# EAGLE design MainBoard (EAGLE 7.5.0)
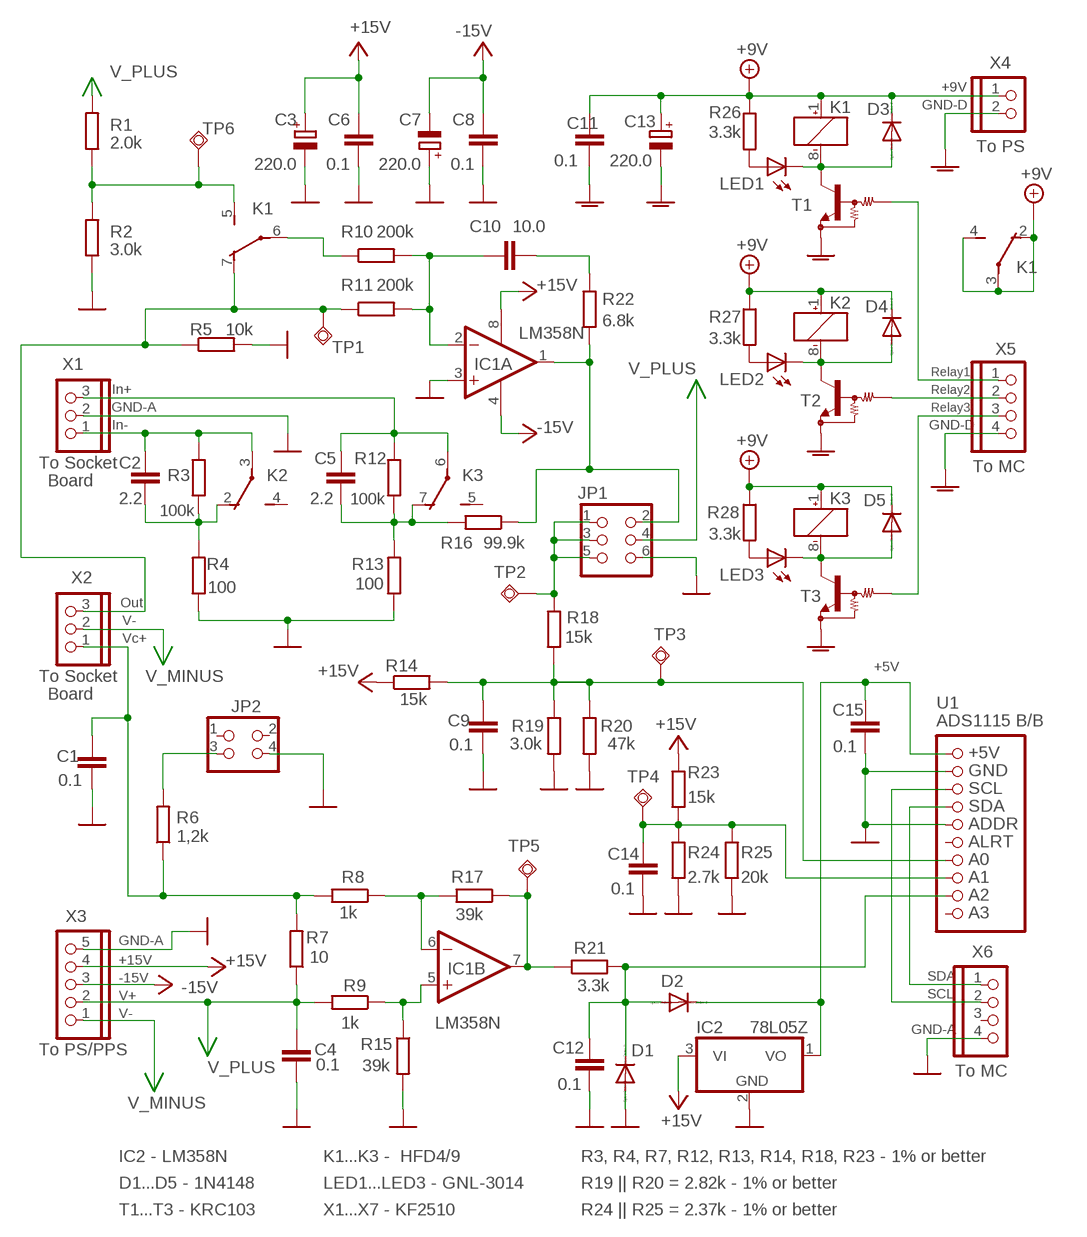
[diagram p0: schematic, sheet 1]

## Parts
C1  0.1  C-EU050-025X075  [C050-025X075]
C2  2.2  C-EU050-025X075  [C050-025X075]
C3  220.0  CPOL-EUE3.5-8  [E3,5-8]
C4  0.1  C-EU075-032X103  [C075-032X103]
C5  2.2  C-EU050-025X075  [C050-025X075]
C6  0.1  C-EU050-025X075  [C050-025X075]
C7  220.0  CPOL-EUE2.5-6  [E2,5-6]
C8  0.1  C-EU050-025X075  [C050-025X075]
C9  0.1  C-EU050-025X075  [C050-025X075]
C10  10.0  C-EU050-025X075  [C050-025X075]
C11  0.1  C-EU050-025X075  [C050-025X075]
C12  0.1  C-EU050-025X075  [C050-025X075]
C13  220.0  CPOL-EUE5-8.5  [E5-8,5]
C14  0.1  C-EU050-025X075  [C050-025X075]
C15  0.1  C-EU050-025X075  [C050-025X075]
D1  1N4148  DIODE-D-5  [D-5]
D2  1N4148  DIODE-D-5  [D-5]
D3  1N4148  DIODE-D-5  [D-5]
D4  1N4148  DIODE-D-5  [D-5]
D5  1N4148  DIODE-D-5  [D-5]
IC1  LM358N  [DIL08]
IC2  78L05Z  [TO92]
JP1  Dupont 2x3  PINHD-2X3  [2X03]
JP2  Dupont 2x2  PINHD-2X2  [2X02]
K1  GQ20009  [GQ]
K2  GQ20009  [GQ]
K3  GQ20009  [GQ]
LED1  GNL-3014  LED3MM  [LED3MM]
LED2  GNL-3014  LED3MM  [LED3MM]
LED3  GNL-3014  LED3MM  [LED3MM]
R1  2.0k  R-EU_0204/7  [0204/7]
R2  3.0k  R-EU_0204/5  [0204/5]
R3  100k  R-EU_0204/5  [0204/5]
R4  100  R-EU_0204/5  [0204/5]
R5  10k  R-EU_0204/7  [0204/7]
R6  1,2k  R-EU_0204/5  [0204/5]
R7  10  R-EU_0204/5  [0204/5]
R8  1k  R-EU_0204/5  [0204/5]
R9  1k  R-EU_0204/5  [0204/5]
R10  200k  R-EU_0204/5  [0204/5]
R11  200k  R-EU_0204/5  [0204/5]
R12  100k  R-EU_0204/5  [0204/5]
R13  100  R-EU_0204/5  [0204/5]
R14  15k  R-EU_0204/5  [0204/5]
R15  39k  R-EU_0204/5  [0204/5]
R16  99.9k  R-EU_0204/7  [0204/7]
R17  39k  R-EU_0204/5  [0204/5]
R18  15k  R-EU_0204/7  [0204/7]
R19  3.0k  R-EU_0204/5  [0204/5]
R20  47k  R-EU_0204/5  [0204/5]
R21  3.3k  R-EU_0204/5  [0204/5]
R22  6.8k  R-EU_0204/5  [0204/5]
R23  15k  R-EU_0204/5  [0204/5]
R24  2.7k  R-EU_0204/5  [0204/5]
R25  20k  R-EU_0204/5  [0204/5]
R26  3.3k  R-EU_0204/5  [0204/5]
R27  3.3k  R-EU_0204/5  [0204/5]
R28  3.3k  R-EU_0204/5  [0204/5]
T1  KRC103  -NPN_DRIVER-TO-92  [TO92-ECB]
T2  KRC103  -NPN_DRIVER-TO-92  [TO92-ECB]
T3  KRC103  -NPN_DRIVER-TO-92  [TO92-ECB]
TP1  TPSQPAD1-13  [P1-13]
TP2  TPSQPAD1-13  [P1-13]
TP3  TPSQPAD1-13  [P1-13]
TP4  TPSQPAD1-13  [P1-13]
TP5  TPSQPAD1-13  [P1-13]
TP6  TPSQPAD1-13  [P1-13]
U1  ADS1115 B/B  PINHD-1X10  [1X10]
X1  KF2510-3P  PINHD-1X3  [1X03]
X2  KF2510-3P  PINHD-1X3  [1X03]
X3  KF2510-5P  PINHD-1X5  [1X05]
X4  KF2510-2P  PINHD-1X2  [1X02]
X5  KF2510-4P  PINHD-1X4  [1X04]
X6  KF2510-4P  PINHD-1X4  [1X04]

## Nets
+5V: C15.2 D2.C IC2.1(VO) U1.1
+9V: C11.2 C13.+ D3.C D4.C D5.C K1.1(1:+) K1.2(2:O) K1.3(2:P) K1.4(2:S) K2.1(1:+) K3.1(1:+) R26.1 R27.1 R28.1 X4.1
ADC_A0: C9.2 R14.2 R18.2 R19.1 R20.1 TP3.TP U1.7
GND-A: C1.1 C3.- C4.1 C6.1 C7.+ C8.1 C9.1 C12.1 C14.1 C15.1 D1.A IC1.3(A:+IN) IC2.2(GND) JP1.6 JP2.4 R2.1 R4.1 R5.2 R13.1 R15.2 R19.2 R20.2 R24.2 R25.2 U1.2 U1.5 X1.2 X3.5 X6.4 ; supply symbol labelled GND
GND-D: C11.1 C13.- T1.E T2.E T3.E X4.2 X5.4 ; supply symbol labelled GNDA
N$1: C2.1 K2.2(2:O) R3.1 R4.2
N$2: C5.1 K3.7(3:O) R12.1 R13.2 R16.2
N$3: C2.2 K2.3(2:P) R3.2 X1.1
N$4: C5.2 K3.6(3:P) R12.2 X1.3
N$5: C14.2 R23.2 R24.1 R25.1 TP4.TP U1.8
N$6: D3.A K1.8(1:-) LED1.K(C) T1.C
N$7: T2.B X5.2
N$9: K1.6(3:P) R10.1
N$11: C10.1 IC1.2(A:-IN) R10.2 R11.2
N$12: C10.2 R22.1
N$13: D4.A K2.8(1:-) LED2.K(C) T2.C
N$14: IC1.7(B:OUT) R17.1 R21.1 TP5.TP
N$15: LED3.A R28.2
N$16: D5.A K3.8(1:-) LED3.K(C) T3.C
N$17: LED2.A R27.2
N$18: JP2.3 R6.2
N$19: K1.5(3:S) R1.1 R2.2 TP6.TP
N$22: T1.B X5.1
N$23: T3.B X5.3
N$24: IC1.6(B:-IN) R8.1 R17.2
N$25: LED1.A R26.2
N$26: IC1.5(B:+IN) R9.1 R15.1
N$27: IC1.1(A:OUT) JP1.2 R16.1 R22.2
N$28: U1.3 X6.2
N$29: U1.4 X6.1
N$31: JP1.1 JP1.3 JP1.5 R18.1 TP2.TP
N$35: C12.2 D1.C D2.A R21.2 U1.9
OUT: K1.7(3:O) R5.1 R11.1 TP1.TP X2.3
V+: C3.+ C6.2 IC1.8(P:V+) IC2.3(VI) R14.1 R23.1 X3.4 ; supply symbol labelled +15V
V-: C7.- C8.2 IC1.4(P:V-) X3.3 ; supply symbol labelled -15V
V_MINUS: X2.2 X3.1
V_PLUS: C4.2 JP1.4 R1.2 R7.1 R9.2 X3.2
VC_PLUS: C1.2 R6.1 R7.2 R8.2 X2.1
Unconnected: JP2.1 JP2.2 K2.4(2:S) K2.5(3:S) K2.6(3:P) K2.7(3:O) K3.2(2:O) K3.3(2:P) K3.4(2:S) K3.5(3:S) U1.6 U1.10 X6.3

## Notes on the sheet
- +9V
- GND-D
- To PS
- Relay1
- In+ | Relay2
- GND-A | Relay3
- In- | GND-D
- To MC
- To Socket
- Board
- Out
- V-
- Vc+
- +5V
- To Socket
- Board
- +5V
- GND
- SCL
- SDA
- ADDR
- ALRT
- A0
- A1
- A2
- A3
- GND-A
- +15V
- -15V | SDA
- V+ | SCL
- V-
- GND-A
- To PS/PPS
- To MC
- IC2 - LM358N | K1...K3 -  HFD4/9 | R3, R4, R7, R12, R13, R14, R18, R23 - 1% or better
- D1...D5 - 1N4148 | LED1...LED3 - GNL-3014 | R19 || R20 = 2.82k - 1% or better
- T1...T3 - KRC103 | X1...X7 - KF2510 | R24 || R25 = 2.37k - 1% or better

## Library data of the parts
C1 C2 C4-C6 C8-C12 C14 C15 = resistor:C-EU: CAPACITOR, European symbol
C3 C7 C13 = resistor:CPOL-EU: POLARIZED CAPACITOR, European symbol
D1-D5 = diode:DIODE-: DIODE
IC1 = linear:LM358: OP AMP also LM158; LM258; LM2904 Source: http://cache.national.com/ds/LM/LM158.pdf
IC2 = linear:78*: Positive VOLTAGE REGULATOR Source: http://cache.national.com/ds/LM/LM78L05.pdf http://www.fairchildsemi.com/ds/LM/LM7805.pdf
JP1 = pinhead:PINHD-2X3: PIN HEADER
JP2 = pinhead:PINHD-2X2: PIN HEADER
K1-K3 = relay:GQ?*: ULTRA-SMALL PACKAGE FLAT POLARIZED RELAY NAiS Source: http://www.mew-europe.com/.. en_ds_61008_0000.pdf; MF: AROMAT/ MATSUSHITA; MPN: AGQ20009; OC_FARNELL: unknown; OC_NEWARK: 10C3361
LED1-LED3 = led:LED: LED
R1-R28 = resistor:R-EU_: RESISTOR, European symbol
T1-T3 = transistor-neu-to92:*-NPN_DRIVER-: NPN Bias Resistor Transistor
TP1-TP6 = testpad:TPSQ: Test pad
U1 = pinhead:PINHD-1X10: PIN HEADER
X1 X2 = pinhead:PINHD-1X3: PIN HEADER
X3 = pinhead:PINHD-1X5: PIN HEADER
X4 = pinhead:PINHD-1X2: PIN HEADER
X5 X6 = pinhead:PINHD-1X4: PIN HEADER

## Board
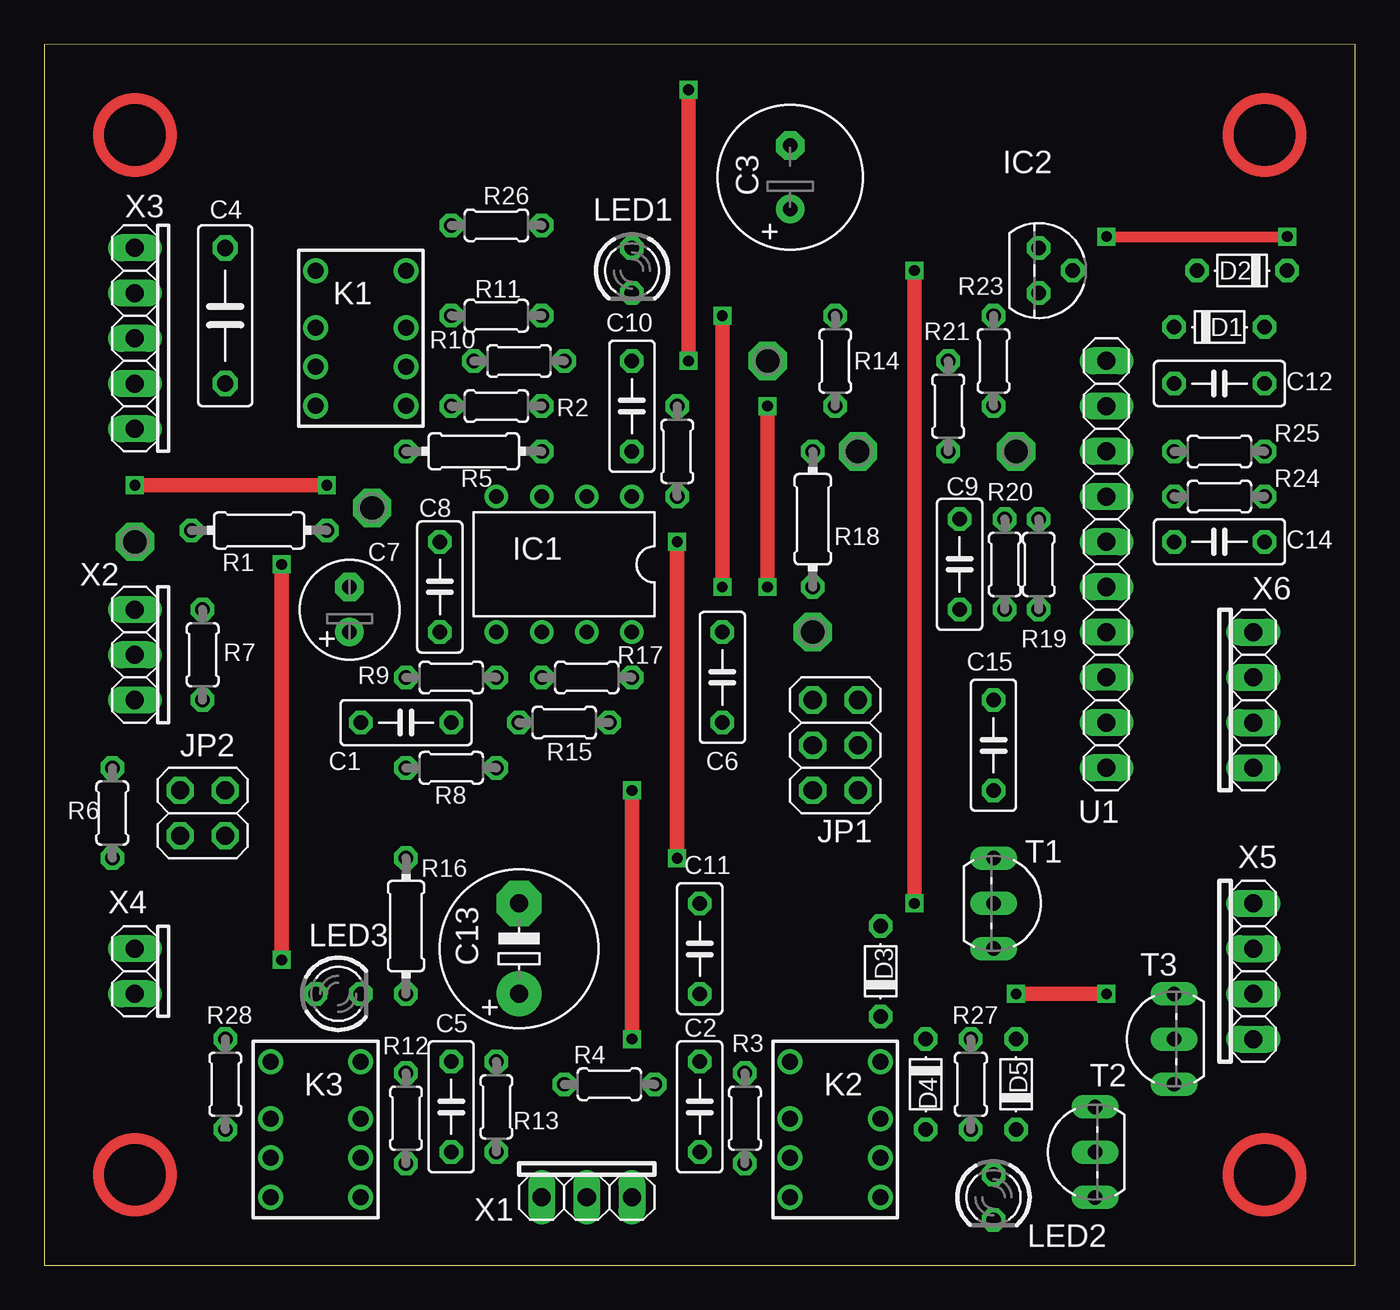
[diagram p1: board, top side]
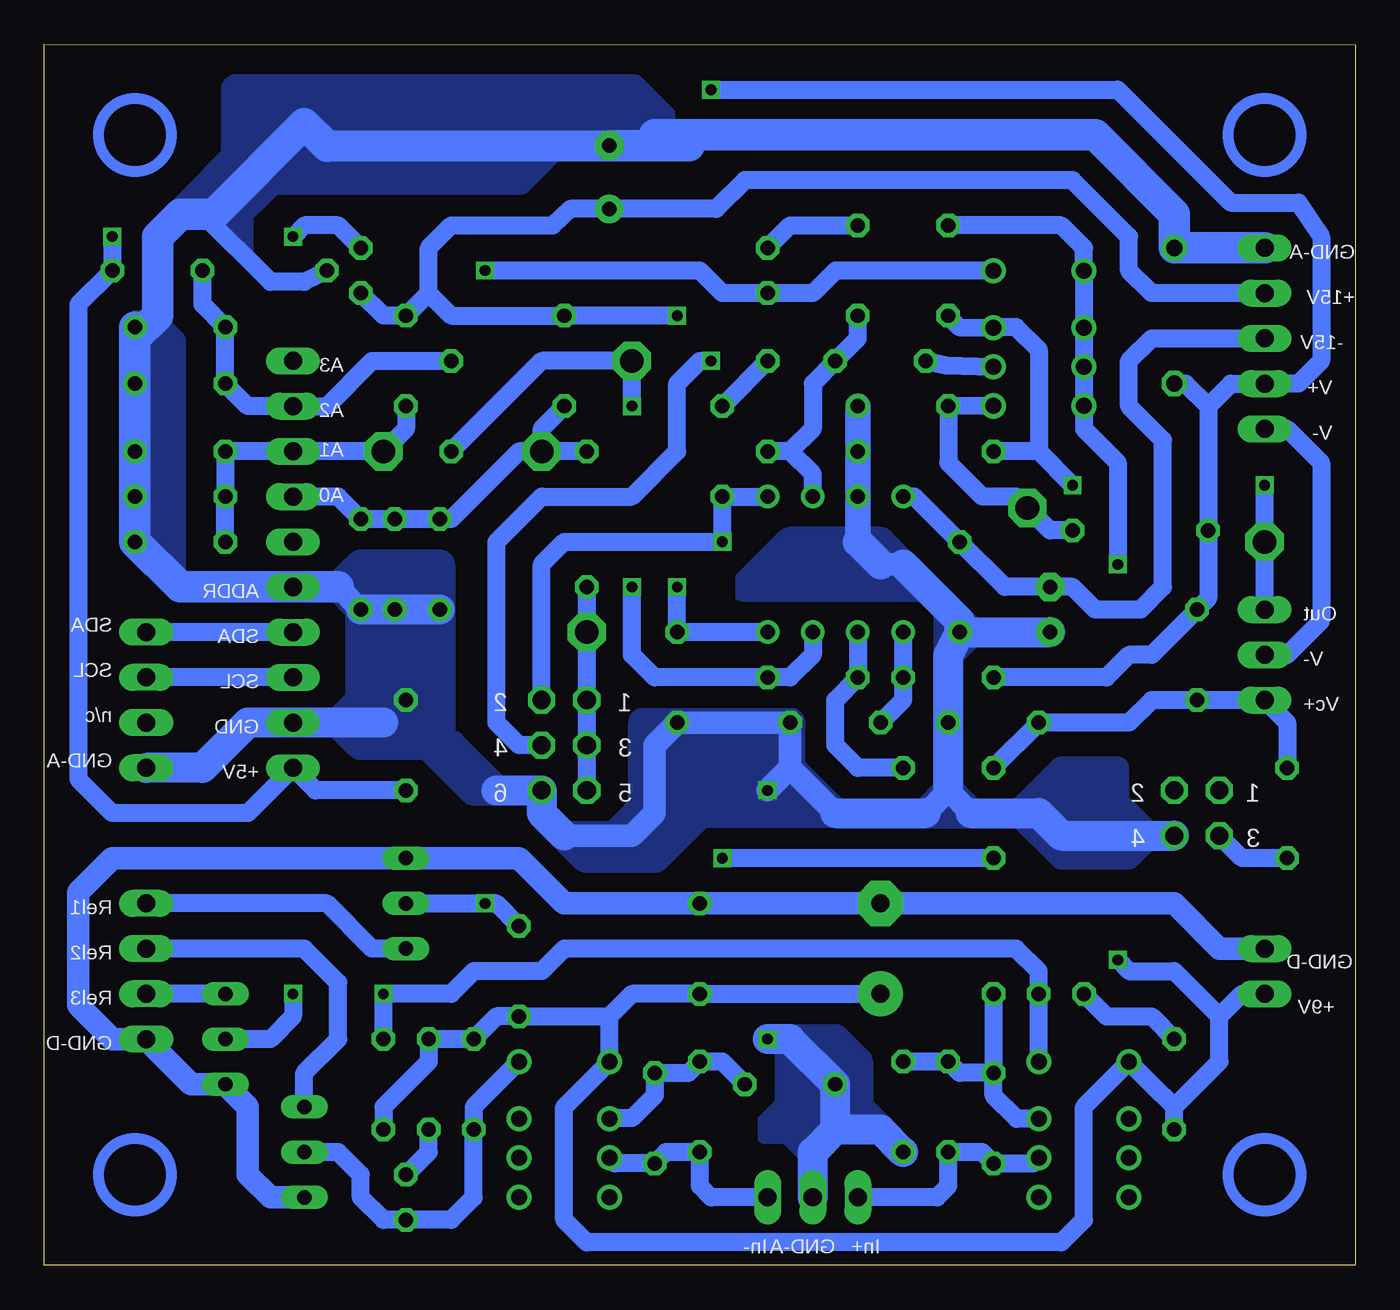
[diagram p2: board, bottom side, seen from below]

Size 73.66 x 68.58 mm. Coordinates in mm from the lower left corner, seen from the top.
Outline: 0,0 73.66,0 73.66,68.58 0,68.57 0,0
Copper layers (1*16): Top 0.035mm / dielectric 1.5mm / Bottom 0.035mm
Design rules "default *": minimum track width 10mil, minimum drill 10mil, track to track 8mil, track to pad 8mil, pad to pad 8mil, via to via 8mil, smd to smd 0mil, copper to edge 0mil, drill to drill 0mil, minimum pad ring 10mil, minimum via ring 8mil, stop-mask expansion 4mil, vias tented up to drill 0mil, thermal gap 10mil

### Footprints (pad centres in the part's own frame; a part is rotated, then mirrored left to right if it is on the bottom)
C050-025X075 = drill 0.813 octagon: 1 -2.54,0; 2 2.54,0
E3,5-8 = drill 0.813 pad 1.6: + -1.778,0 | drill 0.813 pad 1.6 octagon: - 1.778,0
C075-032X103 = drill 0.914 octagon: 1 -3.81,0; 2 3.81,0
E2,5-6 = drill 0.813 pad 1.6: + -1.27,0 | drill 0.813 pad 1.6 octagon: - 1.27,0
E5-8,5 = drill 1.016 pad 2.54: + -2.54,0 | drill 1.016 pad 2.54 octagon: - 2.54,0
D-5 = drill 0.813 octagon: A 2.54,0; C -2.54,0
DIL08 = drill 0.813 pad 1.27: 1 -3.81,-3.81; 2 -1.27,-3.81; 3 1.27,-3.81; 4 3.81,-3.81; 5 3.81,3.81; 6 1.27,3.81; 7 -1.27,3.81; 8 -3.81,3.81
TO92 = drill 0.813 octagon: 1 -1.27,0; 2 0,1.905; 3 1.27,0
2X03 = drill 1.016 octagon: 1 -2.54,-1.27; 2 -2.54,1.27; 3 0,-1.27; 4 0,1.27; 5 2.54,-1.27; 6 2.54,1.27
2X02 = drill 1.016 octagon: 1 -1.27,-1.27; 2 -1.27,1.27; 3 1.27,-1.27; 4 1.27,1.27
GQ = drill 0.9: 1 -3.8,-2.54; 2 -0.6,-2.54; 3 1.6,-2.54; 4 3.8,-2.54; 5 3.8,2.54; 6 1.6,2.54; 7 -0.6,2.54; 8 -3.8,2.54
LED3MM = drill 0.813 octagon: A -1.27,0; K 1.27,0
0204/7 = drill 0.813 octagon: 1 -3.81,0; 2 3.81,0
0204/5 = drill 0.813 octagon: 1 -2.54,0; 2 2.54,0
TO92-ECB = drill 0.813 long: B 2.54,0; C 0,0; E -2.54,0
P1-13 = drill 1.321 pad 2.159 octagon: TP 0,0
1X10 = drill 1.016 long: 1 -11.43,0; 2 -8.89,0; 3 -6.35,0; 4 -3.81,0; 5 -1.27,0; 6 1.27,0; 7 3.81,0; 8 6.35,0; 9 8.89,0; 10 11.43,0
1X03 = drill 1.016 long: 1 -2.54,0; 2 0,0; 3 2.54,0
1X05 = drill 1.016 long: 1 -5.08,0; 2 -2.54,0; 3 0,0; 4 2.54,0; 5 5.08,0
1X02 = drill 1.016 long: 1 -1.27,0; 2 1.27,0
1X04 = drill 1.016 long: 1 -3.81,0; 2 -1.27,0; 3 1.27,0; 4 3.81,0

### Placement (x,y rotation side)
C1  20.32,30.48 180 top
C2  36.83,8.89 270 top
C3  41.91,61.12 90 top
C4  10.16,53.34 270 top
C5  22.86,8.89 270 top
C6  38.1,33.02 90 top
C7  17.14,36.83 90 top
C8  22.23,38.1 90 top
C9  51.44,39.37 90 top
C10  33.02,48.26 90 top
C11  36.83,17.78 270 top
C12  66.04,49.53 180 top
C13  26.67,17.78 90 top
C14  66.04,40.64 180 top
C15  53.34,29.21 270 top
D1  66.04,52.7 0 top
D2  67.31,55.88 180 top
D3  46.99,16.51 90 top
D4  49.53,10.16 270 top
D5  54.61,10.16 90 top
IC1  29.21,39.37 180 top
IC2  55.88,55.88 270 top
JP1  44.45,29.21 270 top
JP2  8.89,25.4 270 top
K1  17.78,52.07 270 top
K2  44.45,7.62 270 top
K3  15.24,7.62 270 top
LED1  33.02,55.88 270 top
LED2  53.34,3.81 270 top
LED3  16.51,15.24 0 top
R1  12.06,41.27 180 top
R2  25.4,48.26 180 top
R3  39.37,8.26 270 top
R4  31.75,10.16 0 top
R5  24.13,45.72 0 top
R6  3.81,25.4 270 top
R7  8.89,34.29 270 top
R8  22.86,27.94 180 top
R9  22.86,33.02 180 top
R10  26.67,50.8 0 top
R11  25.4,53.34 0 top
R12  20.32,8.26 270 top
R13  25.4,8.89 90 top
R14  44.45,50.8 270 top
R15  29.21,30.48 0 top
R16  20.32,19.05 270 top
R17  30.48,33.02 180 top
R18  43.18,41.91 90 top
R19  55.88,39.37 270 top
R20  53.98,39.37 270 top
R21  50.8,48.26 90 top
R22  35.56,45.72 270 top
R23  53.34,50.8 270 top
R24  66.04,43.18 0 top
R25  66.04,45.72 0 top
R26  25.4,58.42 0 top
R27  52.07,10.16 270 top
R28  10.16,10.16 90 top
T1  53.34,20.32 270 top
T2  59.05,6.35 90 top
T3  63.5,12.7 90 top
TP1  5.08,40.64 0 top
TP2  43.18,35.56 0 top
TP3  45.72,45.72 0 top
TP4  54.61,45.72 0 top
TP5  40.64,50.8 0 top
TP6  18.41,42.55 0 top
U1  59.69,39.37 90 top
X1  30.48,3.81 180 top
X2  5.08,34.29 90 top
X3  5.08,52.07 90 top
X4  5.08,16.51 90 top
X5  67.94,16.51 270 top
X6  67.94,31.75 270 top

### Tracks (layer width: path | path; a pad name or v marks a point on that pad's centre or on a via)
+5V  (via drill 0.6)
  Top 0.61: v59.69,57.78 v69.85,57.78
  Bottom 1.016: C15.2 58.42,26.67 U1.1 62.23,25.4 69.85,25.4 71.75,27.3 71.75,53.98 D2.C v69.85,57.78 | IC2.1 57.15,58.42 59.05,58.42 v59.69,57.78
+9V  (via drill 0.6)
  Top 0.813: v13.34,39.37 v13.34,17.14
  Bottom 1.016: C13.+ C11.2 40.64,15.24 41.91,13.97 | v13.34,39.37 13.34,45.09 15.24,46.99 K1.4 K1.3 K1.2 K1.1 15.24,57.15 16.51,58.42 R26.1 | v13.34,17.14 12.7,16.51 10.16,16.51 7.62,13.97 | 10.16,8.89 11.44,10.16 K3.1 15.23,8.89 15.24,8.89 15.24,2.54 16.51,1.27 43.18,1.27 44.45,2.54 44.45,8.89 44.44,8.89 K2.1 41.91,13.97 | R28.1 10.16,8.89 | 10.16,8.89 7.62,11.43 7.62,13.97 | 7.62,13.97 6.35,15.24 X4.1 | 41.91,13.97 D3.C 48.26,13.97 D4.C R27.1 52.07,11.43 54.61,8.89 D5.C
ADC_A0
  Bottom 1.016: U1.7 57.15,43.18 R19.1 R20.1 C9.2 50.8,41.91 46.99,45.72 TP3.TP | R18.2 TP3.TP | TP3.TP 45.72,46.99 R14.2
GND-A  (via drill 0.6)
  Top 0.813: v33.02,12.7 v33.02,26.67
  Bottom 1.016: IC2.2 59.05,55.24 60.96,55.24 64.77,59.05
  Bottom 1.27: 31.75,27.94 R15.2 C6.1 39.37,29.21 39.37,25.4 40.64,24.13 44.45,24.13 | 31.75,27.94 29.21,25.4 | 24.13,25.4 22.86,26.67 21.59,25.4 | 25.4,39.37 26.67,39.37 | v33.02,26.67 31.75,27.94 | R19.2 57.15,38.1
  Bottom 1.422: 27.94,40.64 IC1.3 R5.2 R2.1
  Bottom 1.676: X6.4 64.77,27.94 62.23,30.48 U1.2 54.61,30.48 | 29.21,25.4 24.13,25.4 | 22.86,26.67 C1.1 22.86,34.29 C8.1 | 21.59,25.4 17.78,25.4 16.51,24.13 JP2.4 | 26.67,39.37 27.94,40.64 | 44.45,24.13 45.72,25.4 JP1.6 48.26,26.67 | C8.1 22.23,36.2 25.4,39.37 | C8.1 C7.+ | C9.1 R20.2 R19.2 | X1.2 30.48,6.35 29.21,7.62 | 29.21,7.62 R4.1 31.75,12.7 v33.02,12.7 | 29.21,7.62 26.67,7.62 R13.1
  Bottom 1.778: X3.5 C4.1 10.16,59.05 14.61,63.5 39.37,63.5 37.43,62.9 C3.- 57.78,62.87 59.05,64.14 64.14,59.05 64.77,59.05 66.04,59.05 67.31,57.78 67.31,53.34 68.58,52.07 | 57.15,38.1 U1.5 66.04,38.1 C14.1 R24.2 R25.2 C12.1 68.58,52.07 | D1.A 68.58,52.07
  pour Bottom (no thermals): 31.75,27.94 34.29,25.4 36.83,25.4 39.37,22.86 43.18,22.86 44.45,24.13 40.64,24.13 40.01,24.77 40.01,30.48 31.75,30.48
  pour Bottom (no thermals): 29.21,25.4 34.29,25.4 34.29,27.94 31.75,27.94
  pour Bottom: 39.37,26.67 41.91,24.13 39.37,24.13
  pour Bottom (no thermals): 24.13,38.1 26.67,40.64 31.75,40.64 34.29,38.1
  pour Bottom (no thermals): 51.44,29.21 55.88,29.21 57.15,30.48 55.88,31.75 55.88,36.83 57.15,38.1 55.88,39.37 51.44,39.37
  pour Bottom: 52.07,29.21 49.53,26.67 48.26,26.67 50.8,29.21
  pour Bottom: 21.59,35.56 22.86,36.83 22.86,34.29
  pour Bottom (no thermals): 21.59,25.4 22.86,26.67 24.13,25.4
  pour Bottom (no thermals): 38.73,64.14 40.64,66.04 62.87,66.04 62.87,61.59
  pour Bottom (no thermals): 21.59,35.56 22.86,36.83 22.86,34.29
  pour Bottom (no thermals): 44.45,63.5 46.99,60.96 61.59,60.96 61.59,61.59 58.42,64.77 45.72,64.77
  pour Bottom (no thermals): 59.69,60.96 62.23,60.96 63.5,59.69
  pour Bottom (no thermals): 67.31,53.34 66.04,52.07 66.04,38.1 68.58,40.64 68.58,53.34
  pour Bottom (no thermals): 60.96,62.23 64.14,59.05 66.67,59.05 62.23,63.5
  pour Bottom (no thermals): 62.23,60.96 62.23,56.52 64.77,59.05 62.87,60.96
  pour Bottom (no thermals): 60.96,60.96 63.5,58.42 63.5,60.96
  pour Bottom (no thermals): 26.67,7.62 33.02,7.62 31.75,8.89 31.75,12.7 29.21,12.7 27.94,11.43 27.94,8.89
  pour Bottom (no thermals): 30.48,6.35 31.75,7.62 29.21,10.16 27.94,8.89
  pour Bottom (no thermals): 12.7,22.86 11.43,24.13 13.34,26.04 13.34,27.94 16.51,27.94 19.05,25.4 16.51,22.86
GND-D
  Bottom 1.27: T2.E 60.96,3.81 62.23,5.08 62.23,8.89 T3.E 65.41,10.16 X5.4 69.85,12.7 71.75,14.61 71.75,20.95 69.85,22.86 T1.E 46.99,22.86 44.45,20.32 C11.1 C13.- 10.16,20.32 7.62,17.78 X4.2
N$1
  Bottom 1.016: K2.2 41.88,8.26 40.64,8.26 39.37,9.53 R3.1 37.47,10.79 C2.1 35.56,11.43 R4.2
N$2
  Bottom 1.016: R13.2 C5.1 22.23,10.79 R12.1 | R16.2 R12.1 | K3.7 19.02,8.22 20.32,9.53 R12.1
N$3
  Bottom 1.016: K2.3 41.6,5.71 R3.2 38.73,6.35 C2.2 36.83,4.45 36.2,3.81 X1.1
N$4
  Bottom 1.016: K3.6 18.09,5.71 R12.2 20.95,6.35 C5.2 22.86,4.45 23.5,3.81 X1.3
N$5
  Bottom 1.016: C14.2 R24.1 R25.1 U1.8 TP4.TP 53.34,46.99 R23.2
N$6  (via drill 0.6)
  Top 0.813: v48.9,20.32 v48.9,55.88
  Bottom 1.016: T1.C v48.9,20.32 48.26,20.32 D3.A | v48.9,55.88 36.83,55.88 35.56,54.61 LED1.K 30.48,54.61 29.2,55.87 K1.8
N$7
  Bottom 1.016: X5.2 59.05,17.78 57.15,15.88 57.15,12.7 59.05,10.79 T2.B
N$9
  Bottom 1.016: R10.1 22.99,50.55 K1.6
N$11
  Bottom 1.016: IC1.2 30.48,44.45 31.75,45.72 | 31.75,45.72 C10.1 | R11.2 27.94,52.07 R10.2 30.48,49.53 30.48,46.99 31.75,45.72
N$12
  Bottom 1.016: C10.2 R22.1
N$13
  Bottom 1.016: T2.C 57.15,6.35 55.88,5.08 55.88,3.81 54.61,2.54 LED2.K 50.8,2.54 49.53,3.81 D4.A 49.53,8.89 K2.8
N$14  (via drill 0.6)
  Top 0.813: v40.64,38.1 v40.64,48.26
  Bottom 1.016: v40.64,38.1 40.64,34.29 39.37,33.02 R17.1 31.75,33.02 30.48,34.29 IC1.7 | v40.64,48.26 TP5.TP 45.72,50.8 R21.1
N$15
  Bottom 1.016: LED3.A 13.97,13.97 11.43,13.97 R28.2
N$16  (via drill 0.6)
  Top 0.813: v54.61,15.24 v59.69,15.24
  Bottom 1.016: v59.69,15.24 59.69,13.97 60.96,12.7 T3.C | K3.8 LED3.K 17.78,16.51 19.05,17.78 44.45,17.78 45.72,16.51 49.53,16.51 50.8,15.24 v54.61,15.24 D5.A
N$17
  Bottom 1.016: LED2.A 52.07,6.35 R27.2
N$18
  Bottom 1.016: R6.2 6.35,22.86 JP2.3
N$19
  Bottom 1.016: R1.1 17.14,41.27 TP6.TP 19.05,43.18 20.95,43.18 22.86,45.09 R2.2 K1.5
N$22
  Bottom 1.016: T1.B 55.24,17.78 57.78,20.32 X5.1
N$23
  Bottom 1.016: T3.B X5.3
N$24
  Bottom 1.016: IC1.6 R17.2 29.21,31.75 29.21,29.21 27.94,27.94 R8.1
N$25
  Bottom 1.016: LED1.A 31.75,58.42 R26.2
N$26
  Bottom 1.016: IC1.5 R9.1 25.4,31.75 R15.1
N$27  (via drill 0.6)
  Top 0.813: v35.56,22.86 v35.56,40.64
  Bottom 1.016: JP1.2 45.72,39.37 44.45,40.64 v35.56,40.64 R22.2 IC1.1 | R16.1 v35.56,22.86
N$28
  Bottom 1.016: U1.3 X6.2
N$29
  Bottom 1.016: U1.4 X6.1
N$31
  Bottom 1.016: R18.1 TP2.TP JP1.1 JP1.3 JP1.5
N$35
  Bottom 1.016: D2.A 64.77,53.98 D1.C C12.2 62.23,48.26 U1.9 57.78,48.26 55.24,50.8 R21.2
OUT  (via drill 0.6)
  Top 0.813: v5.08,43.81 v15.88,43.81
  Bottom 1.016: R11.1 22.89,53.34 22.26,52.7 22.23,52.7 K1.7 20.29,52.7 19.05,52.7 17.78,51.44 17.78,45.72 | 17.78,45.72 R5.1 | v15.88,43.81 17.78,45.72 | v5.08,43.81 TP1.TP X2.3
V+  (via drill 0.6)
  Top 0.813: v38.1,38.1 v38.1,53.34
  Bottom 1.016: v38.1,53.34 R14.1 50.8,53.34 52.07,54.61 | v38.1,38.1 C6.2 IC1.8 | X3.4 11.43,54.61 12.7,55.88 12.7,57.78 15.88,60.96 34.29,60.96 35.91,59.34 C3.+ 44.1,59.34 45.09,58.42 50.8,58.42 52.07,57.15 52.07,54.61 | 52.07,54.61 R23.1 54.61,53.34 IC2.3
V-
  Bottom 1.016: IC1.4 24.77,43.18 C8.2 19.68,38.1 C7.- 15.88,38.1 14.61,36.83 12.06,36.83 10.79,38.1 10.79,46.35 12.7,48.26 12.7,50.8 11.43,52.07 X3.3
V_MINUS
  Bottom 1.016: X3.1 3.81,46.99 1.91,45.09 1.91,36.2 3.81,34.29 X2.2
V_PLUS  (via drill 0.6)
  Top 0.813: v36.2,50.8 v36.2,66.04
  Bottom 1.016: 8.26,48.26 6.99,49.53 X3.2 3.17,49.53 1.91,50.8 1.91,57.78 3.17,59.69 6.99,59.69 13.34,66.04 v36.2,66.04 | 8.26,48.26 R1.2 8.26,37.47 R7.1 11.43,34.29 12.7,34.29 13.97,33.02 R9.2 | C4.2 9.53,49.53 8.26,48.26 | JP1.4 46.99,29.21 48.26,30.48 48.26,40.64 45.72,43.18 40.64,43.18 38.1,45.72 38.1,49.53 36.83,50.8 v36.2,50.8
VC_PLUS
  Bottom 1.016: R8.2 C1.2 12.7,30.48 11.43,31.75 R7.2 X2.1 3.81,30.48 R6.1
(copper drawn outside any net)
  shapes: Bottom circle x4, Top circle x4

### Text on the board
bNames: GND-A | +15V | -15V | A3 | V+ | A2 | V- | A1 | A0 | ADDR | Out | SDA | SDA | V- | SCL | SCL | Vc+ | 1 | 2 | GND | n/c | 3 | 4 | GND-A | +5V | 1 | 2 | 5 | 6 | 3 | 4 | Rel1 | GND-D | Rel2 | Rel3 | +9V | GND-D | In+ | GND-A | In-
